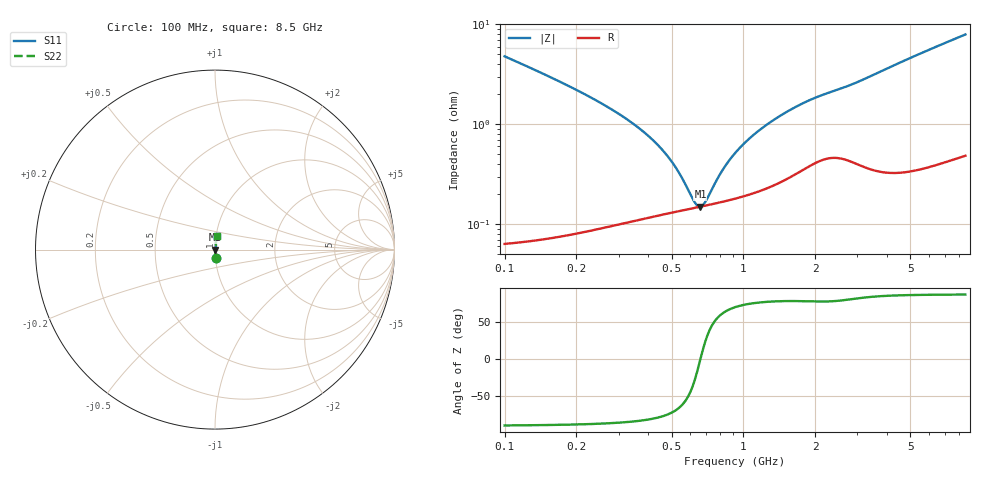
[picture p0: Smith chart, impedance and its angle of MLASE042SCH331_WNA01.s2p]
! MLASE042SCH331_WNA01  S-PARAMETER MODEL  ( General Type )
! Model Generated by TAIYO YUDEN Corporation (http://www.ty-top.com)
! Version 1.0
! TAIYO YUDEN Control No. 180301
! Copyright(c) 2018 TAIYO YUDEN CO.,LTD. All Rights Reserved.
! Product Description (link to TY-COMPAS)
! https://ds.yuden.co.jp/TYCOMPAS/or/detail?pn=MLASE042SCH331JWNA01&u=M
! Products Name : Multilayer Ceramic Capacitors
! Characteristics :
!  Capacitance : 330 pF , Rated Voltage : 16V , TCC : CH / C0H
!  Case Size : 0.4 x 0.2 / 0.016 x 0.008 [mm/inch] , Thickness : 0.2 / 0.008 [mm/inch]
!  (Conditions: Temperature = 25 degC , DC Bias Current/Voltage = 0A / 0V)
! External Node Assignments :
!  1  o---| |---o  2
! GND o---------o GND
! Frequency Range : 100MHz  -  8500MHz  [ 401 STEP ]
# MHz S RI R 50
! Freq[MHz].  S11 Real  S11 Imag  S21 Real  S21 Imag  S12 Real  S12 Imag  S22 Real  S22 Imag
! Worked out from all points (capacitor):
!   401 points, 100 MHz to 8.5 GHz, reference 50 ohm
!   read as one part in series: C = 326 pF near 102.2 MHz
!   lowest |Z| = 150 mohm at 660.7 MHz (marker M1)
!   series resonance near 660.7 MHz, so ESL is about 180 pH
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100  0.00291 -0.0477  0.9971 0.0477  0.9971 0.0477  0.00291 -0.0477
144.2703  0.00174 -0.0321  0.9983 0.0321  0.9983 0.0321  0.00174 -0.0321
196.8958  0.0013 -0.0224  0.9987 0.0224  0.9987 0.0224  0.0013 -0.0224
452.9001  0.00127 -0.00555  0.9987 0.00555  0.9987 0.00555  0.00127 -0.00555
523.2492  0.00134 -0.00336  0.9987 0.00336  0.9987 0.00336  0.00134 -0.00336
618.1043  0.00145 -0.00095  0.9986 0.00095  0.9986 0.00095  0.00145 -0.00095
639.0464  0.00147 -0.000474  0.9985 0.000474  0.9985 0.000474  0.00147 -0.000474
660.6981  0.0015 5.9e-08  0.9985 -5.9e-08  0.9985 -5.9e-08  0.0015 5.9e-08
690.7124  0.00153 0.000631  0.9985 -0.000631  0.9985 -0.000631  0.00153 0.000631
771.8496  0.00163 0.00221  0.9984 -0.00221  0.9984 -0.00221  0.00163 0.00221
834.2525  0.0017 0.00333  0.9983 -0.00333  0.9983 -0.00333  0.0017 0.00333
901.7006  0.00179 0.00447  0.9982 -0.00447  0.9982 -0.00447  0.00179 0.00447
974.6018  0.00189 0.00563  0.9981 -0.00563  0.9981 -0.00563  0.00189 0.00563
1203.579  0.00227 0.00894  0.9977 -0.00894  0.9977 -0.00894  0.00227 0.00894
1502.954  0.00295 0.0127  0.9971 -0.0127  0.9971 -0.0127  0.00295 0.0127
1755.801  0.00367 0.0156  0.9963 -0.0156  0.9963 -0.0156  0.00367 0.0156
2028.529  0.00447 0.0181  0.9955 -0.0181  0.9955 -0.0181  0.00447 0.0181
2926.566  0.0047 0.0252  0.9953 -0.0252  0.9953 -0.0252  0.0047 0.0252
4317.005  0.00477 0.0389  0.9952 -0.0389  0.9952 -0.0389  0.00477 0.0389
5762.285  0.00643 0.0528  0.9936 -0.0528  0.9936 -0.0528  0.00643 0.0528
7116.102  0.00851 0.0654  0.9915 -0.0654  0.9915 -0.0654  0.00851 0.0654
8500  0.0109 0.0778  0.9891 -0.0778  0.9891 -0.0778  0.0109 0.0778
